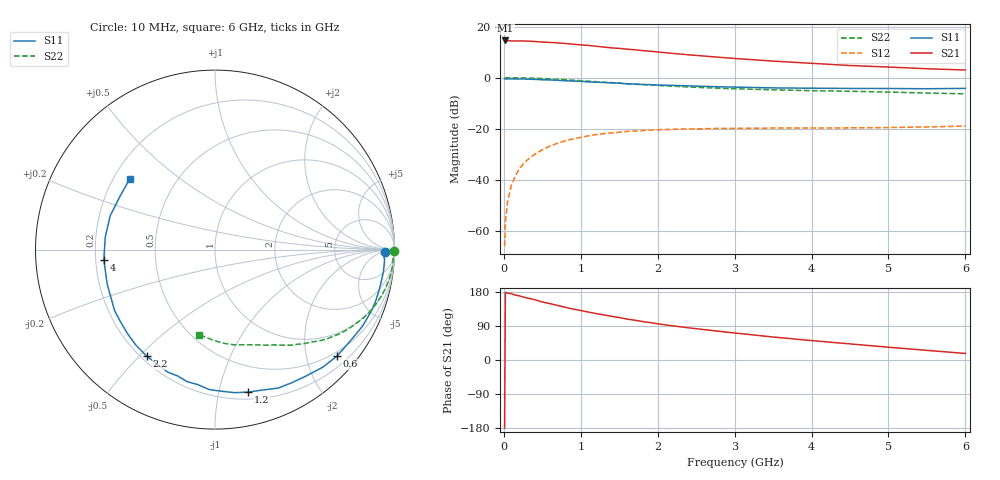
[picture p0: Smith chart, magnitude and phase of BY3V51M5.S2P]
! SIEMENS Small Signal Semiconductors
! BFY420
! Si NPN RF SIEGET Grounded Emitter Transistor in MICRO-X
! VCE = 3.5 V  IC = 1.5 mA
! Common Emitter S-Parameters:  October  1996
# GHz  S  MA  R  50
!  f  S11  S21  S12  S22
! GHz  MAG  ANG  MAG  ANG  MAG  ANG  MAG  ANG
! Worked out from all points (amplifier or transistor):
!   36 points, 10 MHz to 6 GHz, reference 50 ohm
!   highest |S21| = 14.6 dB at 20 MHz (marker M1)
!   |S21| within 3 dB of that: start of sweep to 1.445 GHz
!   unconditionally stable (mu >= 1): 4.255 GHz to end of sweep
!   at 250 MHz: K = 0.04, MSG = 24.2 dB, |S12| = -33.9 dB
!   at 1.4 GHz: K = 0.23, MSG = 16.7 dB, |S12| = -21.6 dB
!   at 6 GHz: K = 1.29, MAG = 7.8 dB, |S12| = -19.0 dB
!   S11 on the Smith chart (normalised r, x): 10 MHz: 35, -9; 600 MHz: 0.41, -2.61; 1.2 GHz: 0.26, -1.22; 2.2 GHz: 0.22, -0.53; 4 GHz: 0.23, -0.04; 6 GHz: 0.27, +0.34
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0.01  0.9473 -0.8  5.354 -179.5  0.0005 79.6  0.9989 -0.4
0.02  0.9409 -1.6  5.358 178.5  0.0015 85.5  0.9909 -0.6
0.05  0.9467 -3.6  5.27 176.7  0.0039 86.1  0.997 -1.6
0.1  0.9465 -7.2  5.25 174.9  0.008 85.3  0.9933 -3.3
0.15  0.9435 -10.4  5.252 171.2  0.0118 81.3  0.9933 -4.9
0.2  0.9419 -14.0  5.236 169.4  0.0164 82.1  0.9915 -6.5
0.3  0.9372 -20.9  5.199 163.7  0.024 77.6  0.9842 -9.7
0.4  0.9259 -27.5  5.122 159.2  0.0315 73.7  0.9737 -12.9
0.5  0.9092 -34.2  4.984 153.1  0.0388 69.7  0.9609 -15.9
0.6  0.9023 -41.1  4.903 148.7  0.0459 66.2  0.9456 -18.9
0.8  0.8695 -53.7  4.672 139.0  0.0579 58.4  0.9114 -24.6
1.1  0.8248 -71.7  4.283 126.5  0.0725 49.7  0.8543 -32.0
1.2  0.8149 -77.0  4.124 122.5  0.0767 46.8  0.8359 -34.3
1.6  0.7578 -97.4  3.619 108.0  0.0886 36.9  0.7631 -42.0
2  0.7187 -115.1  3.184 95.5  0.0955 29.5  0.7041 -48.4
2.2  0.7049 -122.7  2.985 90.1  0.0971 26.3  0.6817 -51.4
2.8  0.6627 -142.6  2.509 75.7  0.1012 19.6  0.6199 -59.0
3.5  0.6306 -162.3  2.111 60.7  0.1029 14.7  0.5779 -66.7
4  0.6218 -174.9  1.911 51.2  0.1034 12.8  0.556 -72.4
4.5  0.6153 173.5  1.733 42.5  0.1039 11.4  0.5414 -78.5
5.5  0.6069 150.6  1.496 25.4  0.1085 11.1  0.5003 -92.5
6  0.617 140.4  1.411 17.3  0.1124 11.1  0.482 -100.6
